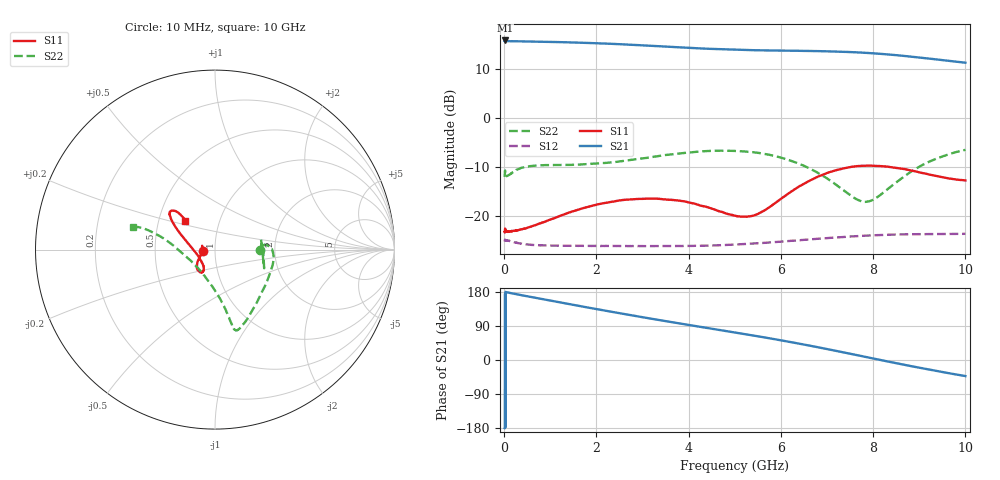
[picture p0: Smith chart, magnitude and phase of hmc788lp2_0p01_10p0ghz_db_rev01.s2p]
! Hittite Microwave Corporation
! 20 Alpha Road
! Chelmsford, MA 01824
! http://www.hittite.com
! Tel: 978-250-3343
! Fax: 978-250-3373
! Device:  HMC788LP2E
! Description: pHEMT GAIN BLOCK MMIC AMPLIFIER
! Frequency:  DC - 10 GHz
! Package:  LP2
! Ports:  2 RF
!  Pad 2 = RF in  = Port 1
!  Pad 3 = Ground
!  Pad 5 = RF out = Port 2
! Voltages:  Vcc = 5.0 Volts
!  Icq = 76 mA;
! Data:  The device was measured using PCB 129549
! Misc:
! Rev. 01
! Date Measured:  Dec-01-2010  KNC
! Date De-embedded: Dec-01-2010  KNC
! Note:
!  Hittite supplies this data as a sample of measured data at the package pin for
!  for this package product. Your particular data for this product may vary.
!  Data was taken at 25 degrees C.
!  Hittite reserves the right to change this data at anytime.
# MHz S MA R 50
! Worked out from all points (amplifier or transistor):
!   2001 points, 10 MHz to 10 GHz, reference 50 ohm
!   highest |S21| = 15.9 dB at 19.99 MHz (marker M1)
!   |S21| within 3 dB of that: start of sweep to 8.498 GHz
!   unconditionally stable (mu >= 1): start of sweep to end of sweep
!   at 1.673 GHz: K = 1.62, MAG = 16.1 dB, |S12| = -26.1 dB
!   at 5.005 GHz: K = 1.64, MAG = 15.2 dB, |S12| = -25.8 dB
!   at 10 GHz: K = 1.53, MAG = 13.2 dB, |S12| = -23.6 dB
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10  0.06889 -172.1  6.126 -179.8  0.05489 1.5  0.2509 -0.7
19.99  0.07459 163.4  6.206 175.0  0.05756 -5.2  0.2928 -20.8
404.605  0.07384 -167.5  6.069 170.3  0.05202 -5.2  0.3129 1.1
799.21  0.0849 -158.5  6.027 161.2  0.05035 -5.3  0.3302 -8.8
1248.76  0.1019 -150.8  5.96 151.1  0.04985 -5.8  0.3326 -18.6
1678.33  0.1191 -144.7  5.882 141.5  0.04969 -6.5  0.3366 -28.4
2112.895  0.1342 -138.5  5.785 132.0  0.04957 -7.3  0.3462 -37.9
2497.51  0.1445 -134.1  5.687 123.6  0.04953 -8.1  0.3611 -46.3
2917.09  0.1495 -128.3  5.556 114.7  0.04949 -8.9  0.3837 -54.3
3341.665  0.1501 -123.2  5.423 105.9  0.04938 -9.6  0.4095 -61.5
4095.91  0.1349 -118.5  5.193 90.6  0.04968 -10.6  0.4499 -70.6
5005  0.1009 -138.0  4.997 72.7  0.05119 -11.8  0.4625 -75.8
5889.115  0.1373 172.4  4.898 54.3  0.05437 -14.3  0.4077 -77.9
6673.33  0.2361 152.2  4.843 36.7  0.05802 -18.3  0.2976 -82.4
7112.89  0.2864 146.5  4.796 26.1  0.06019 -21.3  0.2233 -90.9
7517.485  0.3171 142.6  4.719 16.1  0.06191 -24.2  0.1623 -109.5
7917.085  0.3272 139.6  4.614 6.1  0.06345 -27.5  0.1416 -145.3
8336.665  0.3184 137.0  4.462 -4.4  0.06455 -30.9  0.1918 -176.4
8776.225  0.2952 135.2  4.264 -15.1  0.06522 -34.2  0.2748 169.3
9160.84  0.2695 134.7  4.074 -24.1  0.06545 -36.9  0.3495 164.9
9570.43  0.2463 134.9  3.881 -33.3  0.06571 -39.4  0.4171 163.4
10000  0.2313 135.7  3.678 -42.4  0.06593 -41.4  0.4746 164.8
